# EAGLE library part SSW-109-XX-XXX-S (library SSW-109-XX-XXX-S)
ASSEMBLY, SOCKET STRIP .016 X .031 TAIL. Check prices
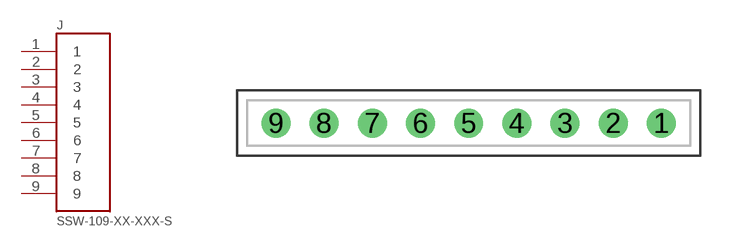
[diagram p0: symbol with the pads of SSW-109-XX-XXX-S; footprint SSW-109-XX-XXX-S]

Designator prefix J

## SSW-109-XX-XXX-S (Availability: Bad; Description: 9 Position Receptacle Connector Surface Mount; MF: Samtec; MP: SSW-109-22-L-S; Package: None; Price: None; Purchase-URL: https://pricing.snapeda.com/search/part/SSW-109-22-L-S/?ref=eda)  [SSW-109-XX-XXX-S]
1  1
2  2
3  3
4  4
5  5
6  6
7  7
8  8
9  9

## Footprint SSW-109-XX-XXX-S (pad centres in mm)
ASSEMBLY, SOCKET STRIP .016 X .031 TAIL.
drill 1.016 pad 1.524: 1 10.16,0; 2 7.62,0; 3 5.08,0; 4 2.54,0; 5 0,0; 6 -2.54,0; 7 -5.08,0; 8 -7.62,0; 9 -10.16,0

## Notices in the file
This work is licensed under a Creative Commons Attribution-ShareAlike 4.0 International License (CC BY-SA) with Design Exception 1.0
